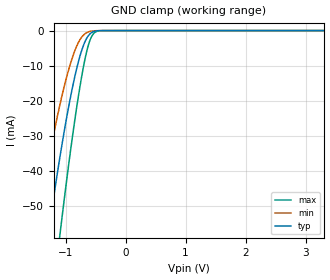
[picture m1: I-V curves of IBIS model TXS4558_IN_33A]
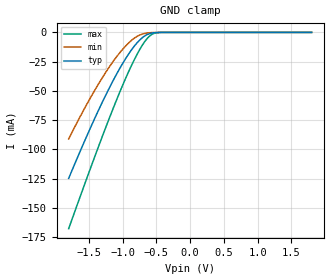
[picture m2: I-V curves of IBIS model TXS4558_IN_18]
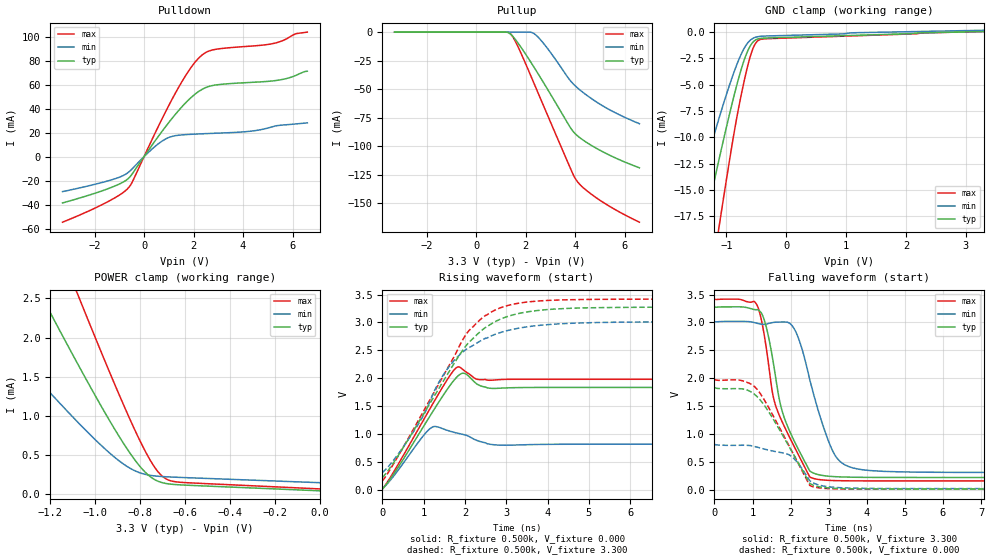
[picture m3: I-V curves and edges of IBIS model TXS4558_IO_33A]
| TEXAS INSTRUMENTS INCORPORATED
| Standard Linear and Logic Group / High Volume Linear
| IBIS Model of TXS4558RUK
| SIM
| This file contains package information for the following:
|  TSSOP 12-pin (PW) package as [Component] TXS4558RUK_PW
| This device can be powered at the following Vccs:
|  3.3 volt Vcc
|  1.8 volt Vcc
| This file provides unique models under the [Model Selector] for each Vcc.
| For operation at a specific Vcc, select the appropriate model after each
| [Model Selector] keyword.
[IBIS Ver]   4.0
[Comment char]  |_char
[File Name]   txs4558.ibs
[File Rev]   1.0 | A2
[Date]   July 20, 2011
[Source]   Data created from TI-SPICE simulations at TI-SLL/HVL.
   The following is an IBIS list for the TXS4558RUK.
   Please contact sllibis@ti.com with questions and
   comments concerning SLL IBIS models.
[Notes]   Revision_History:
   1.0 July 20, 2011
##notes##|
[Disclaimer]
| This model is designed as an aid for customers of Texas Instruments.
| TI and its licensors and suppliers make no warranties, either expressed
| or implied, with respect to this  model, including the warranties of
| merchantability or fitness for a particular purpose. The model is
| provided solely on an "as is" basis. The entire risk as to its quality
| and performance is with the customer.
[Copyright]
| (C) Copyright 2011 Texas Instruments Incorporated. All rights reserved.
| Component TXS4558RUK_PW 20-PIN TSSOP
[Component]   TXS4558RUK_PW
[Manufacturer]   Texas Instruments, Inc.
[Package]
|   typ   min   max
R_pkg   6.163e-02   5.570e-02   7.792e-02
L_pkg   6.209e-10   5.120e-10   8.829e-10
C_pkg   2.201e-13   1.699e-13   2.770e-13
[Pin]   signal_name   model_name   R_pin   L_pin   C_pin
1   VSIM2   POWER   6.741e-02   7.698e-10   2.709e-13
2   VCC   POWER   6.368e-02   5.885e-10   2.480e-13
3   VBAT   POWER   5.617e-02   5.165e-10   1.834e-13
4   VSIM1   POWER   6.741e-02   7.698e-10   2.709e-13
5   SIM1_CLK   TXS4558_OUT   5.570e-02   5.120e-10   2.445e-13
6   SIM1_RST   TXS4558_OUT   5.931e-02   6.876e-10   2.586e-13
7   SIM1_IO   TXS4558_IO   6.291e-02   5.912e-10   1.729e-13
8   IO   TXS4558_IO   5.813e-02   5.411e-10   1.699e-13
9   RST   TXS4558_IN   6.073e-02   7.052e-10   2.631e-13
10   CLK   TXS4558_IN   6.370e-02   6.004e-10   1.874e-13
11   EN1   TXS4558_IN   7.792e-02   8.829e-10   2.770e-13
12   VSEL1   TXS4558_IN   5.269e-02   5.340e-10   1.819e-13
13   CSEL   TXS4558_IN   5.592e-02   5.720e-10   1.769e-13
14   CLKRUN1   TXS4558_IN   5.437e-02   5.921e-10   1.814e-13
15   CLKRUN2   TXS4558_IN   5.592e-02   5.140e-10   1.235e-13
16   VSEL2   TXS4558_IN   5.749e-02   5.056e-10   1.819e-13
17   EN2   TXS4558_IN   7.852e-02   8.829e-10   2.770e-13
18   SIM2_IO   TXS4558_IO   6.351e-02   5.912e-10   1.729e-13
19   SIM2_RST   TXS4558_OUT   5.981e-02   6.876e-10   2.586e-13
20   SIM2_CLK   TXS4558_OUT   5.385e-02   5.120e-10   2.445e-13
| Model TXS4558_IN
[Model Selector]   TXS4558_IN
TXS4558_IN_33A   3.3 volt Vcc
TXS4558_IN_18   1.8 volt Vcc
| Model TXS4558_IO
[Model Selector]   TXS4558_IO
TXS4558_IO_33A   3.3 volt Vcc
TXS4558_IO_18   1.8 volt Vcc
| Model TXS4558_OUT
[Model Selector]   TXS4558_OUT
TXS4558_OUT_33A   3.3 volt Vcc
TXS4558_OUT_18   1.8 volt Vcc
| Models and submodels in the file (6): TXS4558_IN_33A (Input), TXS4558_IN_18 (Input), TXS4558_IO_33A (I/O), TXS4558_IO_18 (I/O), TXS4558_OUT_33A (Output), TXS4558_OUT_18 (Output)
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[Model]   TXS4558_IN_33A
Model_type  Input
Vinl=0.99
Vinh=2.31
| variable   typ   min   max
C_comp   1.24pF   0.89pF   1.46pF
[Temperature Range]   40   100   -40
| Ambient temperature   25   85   -40
[Voltage range]   3.3   3.15   3.45
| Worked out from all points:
|   GND clamp passes 1 mA (typ) near -0.60 V on its own axis
[GND Clamp]
| TXS4558_IN_33A
|   Voltage   I(typ)   I(min)   I(max)
-3.3V     -343.1mA   -283.9mA   -410.2mA
-1.49V    -83.26mA   -57.19mA   -118.2mA
-1.275V   -56.52mA   -36.34mA   -84.95mA
-1.11V    -37.82mA   -22.41mA   -60.55mA
-1.08V    -34.64mA   -20.12mA   -56.27mA
-960mV    -22.79mA   -11.88mA   -39.83mA
-840mV    -12.69mA   -5.488mA   -24.84mA
-740mV    -6.143mA   -2.087mA   -13.97mA
-640mV    -1.976mA   -535.2uA   -5.442mA
-540mV    -341uA     -96.97uA   -1.007mA
-420mV    -19.34uA   -7.931uA   -40.37uA
3.3V      476.5pA    729.2pA    131.1pA
[Model]   TXS4558_IN_18
Model_type  Input
Vinl=0.54
Vinh=1.26
| variable   typ   min   max
C_comp   1.17pF   0.87pF   1.45pF
[Temperature Range]   40   100   -40
| Ambient temperature   25   85   -40
[Voltage range]   1.8   1.65   1.95
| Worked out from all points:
|   GND clamp passes 1 mA (typ) near -0.60 V on its own axis
[GND Clamp]
| TXS4558_IN_18
|   Voltage   I(typ)   I(min)   I(max)
-1.8V     -124.8mA   -91.08mA   -167.8mA
-1.595V   -97.02mA   -68.24mA   -134.9mA
-1.41V    -73.06mA   -49.13mA   -105.7mA
-1.24V    -52.4mA    -33.21mA   -79.67mA
-1.085V   -35.16mA   -20.49mA   -56.98mA
-940mV    -20.97mA   -10.66mA   -37.21mA
-810mV    -10.52mA   -4.264mA   -21.4mA
-690mV    -3.723mA   -1.11mA    -9.312mA
-595mV    -974.9uA   -258.1uA   -2.866mA
-525mV    -247.6uA   -72.91uA   -718.2uA
-420mV    -19.34uA   -7.931uA   -40.37uA
1.8V      182.3pA    324.5pA    63.6pA
[Model]   TXS4558_IO_33A
Model_type  I/O
Vinl=0.99
Vinh=2.31
Enable   Active-Low
Vref =   0
Rref =   500
Cref =   1p
Vmeas =   1.65
| variable   typ   min   max
C_comp   3.56pF   1.07pF   5.96pF
| C_pullup   2.50pF   1.01pF   5.26pF
| C_pulldown   3.12pF   1.43pF   5.84pF
| C_tri-state   3.56pF   1.07pF   5.96pF
[Temperature Range]   40   100   -40
| Ambient temperature   25   85   -40
[Voltage range]   3.3   3.15   3.45
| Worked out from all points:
|   slope of the pulldown table from 0 to 0.495 V, typ, clamps not added: 34 ohm
|   slope of the pullup table from 0 to 0.495 V, typ, clamps not added: 34.3 kohm
|   GND clamp passes 1 mA (typ) near -0.56 V on its own axis
|   POWER clamp passes 1 mA (typ) near -0.95 V on its own axis
|   rising waveform, R_fixture 0.500k, V_fixture 0.000: 20-80 % time 918ps typ, 480ps min, 914ps max; typ from 0.011 V to 1.83 V
|   falling waveform, R_fixture 0.500k, V_fixture 3.300: 20-80 % time 683ps typ, 688ps min, 759ps max; typ from 3.28 V to 0.218 V
|   rising waveform, R_fixture 0.500k, V_fixture 3.300: 20-80 % time 1.56ns typ, 1.37ns min, 1.47ns max; typ from 0.218 V to 3.28 V
|   falling waveform, R_fixture 0.500k, V_fixture 0.000: 20-80 % time 932ps typ, 667ps min, 923ps max; typ from 1.83 V to 0.011 V
[GND Clamp]
| TXS4558_IO_33A
|   Voltage   I(typ)   I(min)   I(max)
-3.3V     -73.09mA   -55.53mA   -103.9mA
-1.635V   -25.68mA   -18.48mA   -38.01mA
-1.375V   -18.66mA   -13.12mA   -27.98mA
-1.325V   -17.33mA   -12.11mA   -26.08mA
-1.135V   -12.4mA    -8.41mA    -18.95mA
-1.105V   -11.64mA   -7.846mA   -17.84mA
-895mV    -6.561mA   -4.157mA   -10.35mA
-775mV    -3.979mA   -2.39mA    -6.604mA
-640mV    -1.752mA   -1.011mA   -3.126mA
-550mV    -927.8uA   -585.9uA   -1.484mA
-375mV    -583uA     -390uA     -656.9uA
3.3V      42.14uA    162.1uA    46.51uA
[POWER Clamp]
| TXS4558_IO_33A
|   Voltage   I(typ)   I(min)   I(max)
-3.3V     14.21mA    8.275mA    19.06mA
-1.61V    4.584mA    2.611mA    6.436mA
-1.57V    4.36mA     2.48mA     6.14mA
-1.245V   2.562mA    1.433mA    3.756mA
-1.22V    2.426mA    1.355mA    3.575mA
-1.085V   1.701mA    941.4uA    2.603mA
-1.065V   1.596mA    882.3uA    2.461mA
-835mV    483.4uA    315.2uA    892.6uA
-755mV    223.8uA    240uA      434.7uA
-695mV    142uA      223.2uA    215.2uA
-615mV    117.1uA    212.5uA    149.7uA
-48.03fV  42.14uA    145.9uA    66.45uA
[Pulldown]
| TXS4558_IO_33A
|   Voltage   I(typ)   I(min)   I(max)
-3.3V     -38.62mA   -29.17mA   -54.71mA
-1.495V   -27.01mA   -20.4mA    -37.89mA
-620mV    -17.81mA   -12.75mA   -25.64mA
325mV     9.794mA    6.478mA    14.56mA
895mV     25.83mA    15.1mA     38.63mA
1.74V     46.28mA    18.51mA    69.74mA
2.365V    56.49mA    19.15mA    85.3mA
2.94V     60.03mA    19.64mA    89.85mA
4.335V    62.08mA    21.35mA    92.41mA
5.22V     63.36mA    25.18mA    94.54mA
6.13V     67.86mA    27.36mA    102.7mA
6.6V      71.41mA    28.27mA    104.1mA
[Pullup]
| TXS4558_IO_33A
|   Voltage   I(typ)   I(min)   I(max)
-3.3V     0A         0A         0A
1.205V    -35.11uA   0A         -158.8nA
1.36V     -1.306mA   0A         -853.4uA
1.675V    -9.144mA   0A         -12.13mA
2.19V     -25.73mA   -88.74uA   -37.42mA
2.395V    -32.76mA   -2.279mA   -47.86mA
2.885V    -50.1mA    -14.38mA   -72.81mA
3.79V     -83.05mA   -42.1mA    -118.4mA
4.045V    -89.89mA   -47.92mA   -129.6mA
4.37V     -95.31mA   -53.7mA    -137.1mA
4.985V    -103.3mA   -62.9mA    -147mA
6.6V      -118.9mA   -80.26mA   -166.5mA
[Ramp]
| TXS4558_IO_33A
| variable   typ   min   max
dV/dt_r   1.25/1.05E-09   0.67/6.58E-10   1.32/1.02E-09
dV/dt_f   1.84/6.84E-10   1.67/6.89E-10   1.96/7.61E-10
R_load = 500
[Rising Waveform]
R_fixture = 0.500k
V_fixture = 0.000
V_fixture_min = 0.000
V_fixture_max = 0.000
C_fixture = 0.000
L_fixture = 0.000
|  time   V(typ)   V(min)   V(max)
0s        11.02mV    17.35mV    8.348mV
360ps     374.6mV    327mV      424.9mV
1.16ns    1.329V     1.098V     1.461V
1.295ns   1.488V     1.132V     1.634V
1.635ns   1.866V     1.049V     2.046V
1.84ns    2.045V     1.009V     2.203V
1.995ns   2.083V     982.6mV    2.127V
2.275ns   1.903V     886.6mV    1.984V
2.6ns     1.819V     815mV      1.962V
25ns      1.833V     815.2mV    1.98V
[Falling Waveform]
R_fixture = 0.500k
V_fixture = 3.300
V_fixture_min = 3.150
V_fixture_max = 3.450
C_fixture = 0.000
L_fixture = 0.000
|  time   V(typ)   V(min)   V(max)
0s        3.28V      3.018V     3.419V
1.035ns   3.233V     2.999V     3.379V
1.23ns    3.173V     2.968V     3.052V
1.62ns    1.957V     3.004V     1.48V
1.795ns   1.37V      3.008V     1.191V
2.125ns   830mV      2.846V     731.3mV
2.67ns    279.7mV    1.548V     189.2mV
3.225ns   230.7mV    558.5mV    161.1mV
4.1ns     219.8mV    341.4mV    156.7mV
25ns      217.6mV    306.7mV    156.1mV
[Rising Waveform]
R_fixture = 0.500k
V_fixture = 3.300
V_fixture_min = 3.150
V_fixture_max = 3.450
C_fixture = 0.000
L_fixture = 0.000
|  time   V(typ)   V(min)   V(max)
0s        217.6mV    306.7mV    156.1mV
330ps     549.2mV    584.6mV    536.2mV
840ps     1.162V     1.139V     1.2V
1.535ns   2.019V     2.124V     2.12V
2.065ns   2.617V     2.534V     2.824V
2.5ns     2.911V     2.717V     3.127V
3.26ns    3.153V     2.891V     3.34V
4.16ns    3.239V     2.969V     3.399V
5.75ns    3.269V     3.004V     3.416V
25ns      3.28V      3.018V     3.419V
[Falling Waveform]
R_fixture = 0.500k
V_fixture = 0.000
V_fixture_min = 0.000
V_fixture_max = 0.000
C_fixture = 0.000
L_fixture = 0.000
|  time   V(typ)   V(min)   V(max)
0s        1.833V     815.2mV    1.98V
680ps     1.81V      795.8mV    1.962V
1.1ns     1.681V     765.9mV    1.815V
1.405ns   1.417V     711.8mV    1.495V
1.98ns    748.6mV    616.3mV    757.9mV
2.2ns     480.9mV    468mV      470.2mV
2.5ns     114.3mV    161.2mV    77.49mV
2.76ns    50.08mV    79.68mV    30.29mV
4.635ns   11.74mV    19.72mV    8.55mV
25ns      11.03mV    17.35mV    8.347mV
